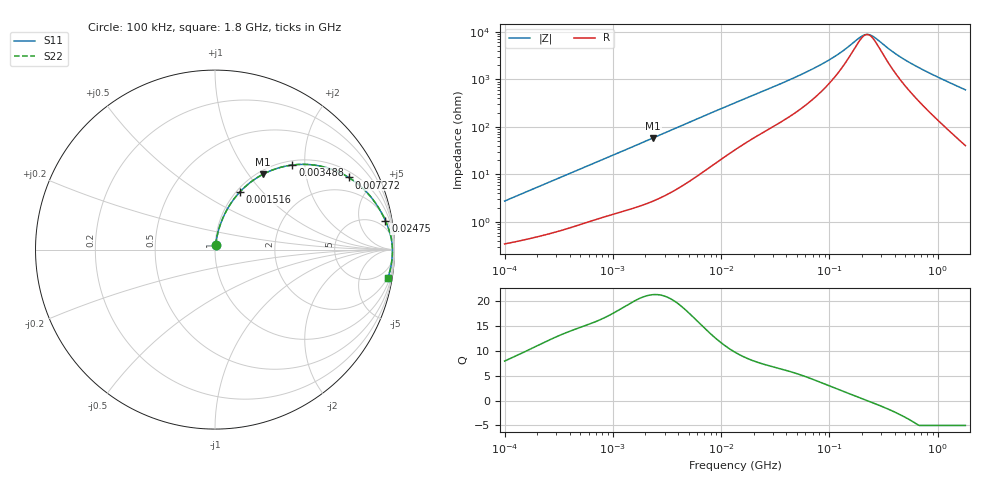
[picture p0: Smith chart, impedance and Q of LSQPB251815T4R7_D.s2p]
! LSQPB251815T4R7_D  S-PARAMETER MODEL  ( General Type )
! Model Generated by TAIYO YUDEN Corporation (http://www.ty-top.com)
! Version 2.0
! TAIYO YUDEN Control No. 110926NG22SB-FKC
! Copyright(c) 2010 TAIYO YUDEN CO.,LTD. All Rights Reserved.
! Product Description (link to TY-COMPAS)
! https://ds.yuden.co.jp/TYCOMPAS/or/detail?pn=LSQPB251815T4R7MD&u=M
! Products Name : Inductors
! Characteristics :
!  Inductance : 4.7 uH , SRF(min) : 150 MHz , DC Resistance(max) : 0.3185 Ohm
!  Rated Current : Saturation :1100 mA , Temp Rise : 750 mA (40 degC)
!  Case Size : 2.5 x 1.8 / 0.098 x 0.071 [mm/inch] , Thickness : 1.5 / 0.06 [mm/inch]
!  (Conditions: Temperature = 25 degC , DC Bias Current/Voltage = 0A / 0V)
! External Node Assignments :
!  1  o---GGG---o  2
! GND o---------o GND
! Frequency Range : 0.1MHz  -  1800MHz  [ 402 STEP ]
# MHz S RI R 50
! Freq[MHz].  S11 Real  S11 Imag  S21 Real  S21 Imag  S12 Real  S12 Imag  S22 Real  S22 Imag
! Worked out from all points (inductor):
!   401 points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, 100 kHz to 1.8 GHz, reference 50 ohm
!   read as one part in series: L = 4.33 uH near 105 kHz
!   highest Q = 21.2 at 2.357 MHz (marker M1), where L = 3.96 uH
!   self-resonance near 222.5 MHz
!   S11 on the Smith chart (normalised r, x): 100 kHz: 1.01, +0.05; 1.516 MHz: 1.04, +0.76; 3.488 MHz: 1.09, +1.73; 7.272 MHz: 1.25, +3.55; 24.75 MHz: 3, +11; 1.8 GHz: 2, -12
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0.1  0.0042 0.0272  0.9958 -0.0272  0.9958 -0.0272  0.0042 0.0272
0.247521  0.00973 0.0649  0.9903 -0.0649  0.9903 -0.0649  0.00973 0.0649
0.516129  0.0262 0.1293  0.9738 -0.1293  0.9738 -0.1293  0.0262 0.1293
0.952166  0.0669 0.2225  0.9331 -0.2225  0.9331 -0.2225  0.0669 0.2225
1.516485  0.1388 0.3213  0.8612 -0.3213  0.8612 -0.3213  0.1388 0.3213
2.356814  0.266 0.4189  0.734 -0.4189  0.734 -0.4189  0.266 0.4189
2.66389  0.3132 0.4408  0.6868 -0.4408  0.6868 -0.4408  0.3132 0.4408
3.487677  0.4311 0.4712  0.5689 -0.4712  0.5689 -0.4712  0.4311 0.4712
4.914404  0.5903 0.4644  0.4097 -0.4644  0.4097 -0.4644  0.5903 0.4644
7.272466  0.7455 0.4018  0.2545 -0.4018  0.2545 -0.4018  0.7455 0.4018
13.41641  0.8888 0.267  0.1112 -0.267  0.1112 -0.267  0.8888 0.267
24.75089  0.9495 0.1607  0.0505 -0.1607  0.0505 -0.1607  0.9495 0.1607
69.24595  0.9829 0.0578  0.0171 -0.0578  0.0171 -0.0578  0.9829 0.0578
113.0207  0.9871 0.0295  0.0129 -0.0295  0.0129 -0.0295  0.9871 0.0295
189.0427  0.9886 0.00664  0.0114 -0.00664  0.0114 -0.00664  0.9886 0.00664
213.6735  0.9887 0.00164  0.0113 -0.00164  0.0113 -0.00164  0.9887 0.00164
229.9669  0.9887 -0.00135  0.0113 0.00135  0.0113 0.00135  0.9887 -0.00135
253.6402  0.9888 -0.00535  0.0112 0.00535  0.0112 0.00535  0.9888 -0.00535
357.3983  0.9885 -0.02  0.0115 0.02  0.0115 0.02  0.9885 -0.02
479.5244  0.9877 -0.0344  0.0123 0.0344  0.0123 0.0344  0.9877 -0.0344
675.6865  0.9859 -0.055  0.0141 0.055  0.0141 0.055  0.9859 -0.055
1800  0.963 -0.158  0.037 0.158  0.037 0.158  0.963 -0.158
